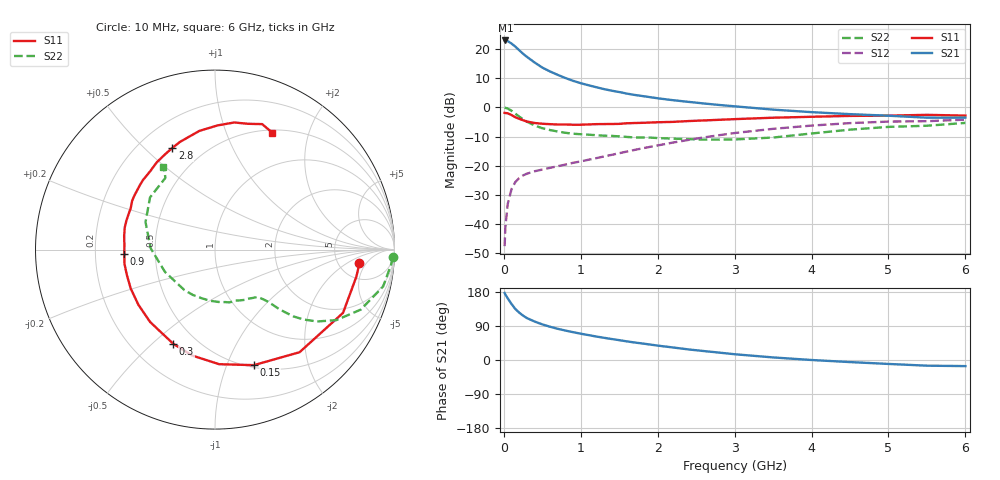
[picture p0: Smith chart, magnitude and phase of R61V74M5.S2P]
! SIEMENS Small Signal Semiconductors
! BFR193
! Si NPN RF Bipolar Junction Transistor in SOT23
! VCE = 1.75 V  IC = 4.5 mA
! Common Emitter S-Parameters:  May  1996
# GHz  S  MA  R  50
!  f  S11  S21  S12  S22
! GHz  MAG  ANG  MAG  ANG  MAG  ANG  MAG  ANG
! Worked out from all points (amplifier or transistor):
!   36 points, 10 MHz to 6 GHz, reference 50 ohm
!   highest |S21| = 23.0 dB at 20 MHz (marker M1)
!   |S21| within 3 dB of that: start of sweep to 185.7 MHz
!   unconditionally stable (mu >= 1): 912.2 MHz to 2.044 GHz
!   at 250 MHz: K = 0.40, MSG = 20.8 dB, |S12| = -23.3 dB
!   at 1.4 GHz: K = 1.08, MAG = 9.3 dB, |S12| = -16.3 dB
!   at 6 GHz: K = 0.98, MSG = 0.3 dB, |S12| = -4.2 dB
!   S11 on the Smith chart (normalised r, x): 10 MHz: 7.89, -3.46; 150 MHz: 0.52, -1.25; 300 MHz: 0.37, -0.58; 900 MHz: 0.33, -0.02; 2.8 GHz: 0.34, +0.61; 6 GHz: 0.54, +1.47
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0.01  0.8083 -5.4  13.94 176.8  0.0042 89.1  0.9918 -2.4
0.02  0.802 -10.8  14.06 172.9  0.0089 84.4  0.9843 -5.0
0.05  0.7957 -26.3  13.72 162.8  0.022 77.0  0.959 -12.4
0.1  0.7409 -50.5  12.42 147.8  0.04 65.8  0.878 -22.4
0.15  0.6792 -71.4  11.01 134.4  0.0528 57.6  0.7814 -30.2
0.2  0.639 -87.9  9.56 125.0  0.0617 52.3  0.6963 -35.1
0.25  0.6037 -102.2  8.314 117.0  0.0685 48.3  0.6283 -38.3
0.3  0.574 -113.9  7.365 110.6  0.0734 46.8  0.5719 -40.5
0.4  0.5416 -131.9  5.894 101.5  0.0806 44.8  0.49 -42.8
0.5  0.526 -144.2  4.822 94.0  0.0863 44.5  0.4413 -43.8
0.6  0.5172 -155.2  4.136 87.8  0.0924 45.3  0.41 -44.7
0.7  0.511 -164.1  3.62 82.3  0.0983 47.1  0.3868 -45.8
0.9  0.5058 -177.4  2.861 73.4  0.1125 50.6  0.3545 -48.3
1.1  0.5119 171.4  2.401 65.7  0.127 53.2  0.3413 -52.2
1.3  0.5193 161.9  2.066 58.7  0.1446 55.3  0.3286 -56.5
1.6  0.5359 149.5  1.727 49.1  0.1755 57.2  0.3126 -65.0
2.2  0.566 129.8  1.331 33.0  0.2505 55.9  0.2923 -86.3
2.8  0.6144 112.7  1.103 19.5  0.3349 49.7  0.2811 -115.8
3.5  0.6671 97.5  0.918 6.8  0.4301 38.5  0.3052 -156.0
4.5  0.7163 81.4  0.768 -5.5  0.5392 21.5  0.4164 158.4
5.5  0.7469 69.4  0.668 -15.0  0.5822 4.5  0.486 124.6
6  0.7251 63.8  0.669 -16.1  0.618 -0.4  0.5434 121.9
